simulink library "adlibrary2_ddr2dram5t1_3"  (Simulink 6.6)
libraries: xbsIndex_r4 x5, adlibrary2_ddr2dram5t1_1 x2

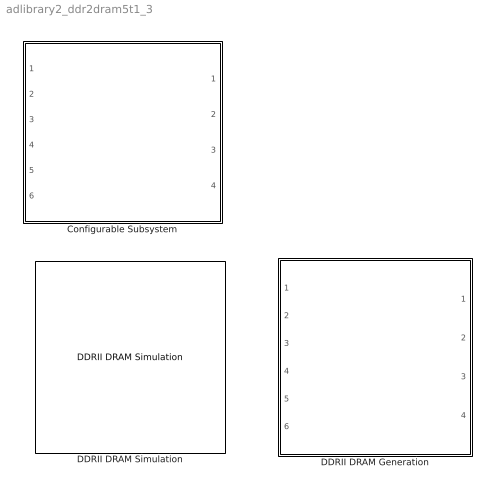
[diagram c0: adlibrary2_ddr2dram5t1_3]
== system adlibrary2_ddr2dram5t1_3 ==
  Configurable Subsystem : Subsystem  BlockChoice=DDRII DRAM Simulation
  DDRII DRAM Generation : Subsystem
  DDRII DRAM Simulation : adlibrary2_ddr2dram5t1_1/DDRII DRAM Simulation  SystemSampleTime=-1

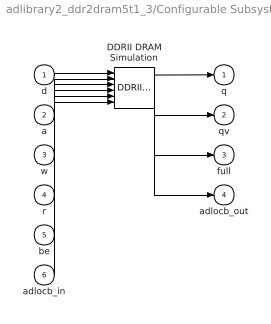
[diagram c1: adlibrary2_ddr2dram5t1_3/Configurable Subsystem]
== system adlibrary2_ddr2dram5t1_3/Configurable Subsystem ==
  d : Inport
  a : Inport  Port=2
  w : Inport  Port=3
  r : Inport  Port=4
  be : Inport  Port=5
  adlocb_in : Inport  Port=6
  DDRII DRAM Simulation : adlibrary2_ddr2dram5t1_1/DDRII DRAM Simulation  SystemSampleTime=-1
  q : Outport
  qv : Outport  Port=2
  full : Outport  Port=3
  adlocb_out : Outport  Port=4
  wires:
  d/1 -> DDRII DRAM Simulation/1
  a/1 -> DDRII DRAM Simulation/2
  w/1 -> DDRII DRAM Simulation/3
  r/1 -> DDRII DRAM Simulation/4
  be/1 -> DDRII DRAM Simulation/5
  adlocb_in/1 -> DDRII DRAM Simulation/6
  DDRII DRAM Simulation/1 -> q/1
  DDRII DRAM Simulation/2 -> qv/1
  DDRII DRAM Simulation/3 -> full/1
  DDRII DRAM Simulation/4 -> adlocb_out/1

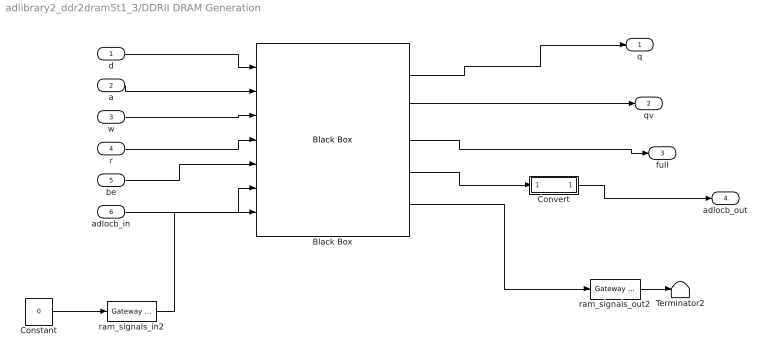
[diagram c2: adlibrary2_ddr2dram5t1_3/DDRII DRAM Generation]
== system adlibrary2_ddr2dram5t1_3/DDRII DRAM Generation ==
  d : Inport
  a : Inport  Port=2
  w : Inport  Port=3
  r : Inport  Port=4
  be : Inport  Port=5
  adlocb_in : Inport  Port=6
  Black Box : xbsIndex_r4/Black Box  init_code=ddr2sdram_v5_config2  sim_method=Inactive  block_type=blackbox2
  Constant : Constant  Value=0
  Convert : Subsystem
  Terminator2 : Terminator
  ram_signals_in2 : xbsIndex_r4/Gateway In  arith_type=Unsigned  n_bits=133  bin_pt=0  quantization="Round  (unbiased: +/- Inf)"  overflow=Saturate  period=ad_get_simulink_period  dbl_ovrd=off  timing_constraint=None  locs_specified=off  LOCs={}  block_type=gatewayin
  ram_signals_out2 : xbsIndex_r4/Gateway Out  hdl_port=on  timing_constraint=None  locs_specified=off  LOCs={}  block_type=gatewayout
  q : Outport
  qv : Outport  Port=2
  full : Outport  Port=3
  adlocb_out : Outport  Port=4
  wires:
  ram_signals_out2/1 -> Terminator2/1
  Constant/1 -> ram_signals_in2/1
  d/1 -> Black Box/1
  a/1 -> Black Box/2
  w/1 -> Black Box/3
  r/1 -> Black Box/4
  be/1 -> Black Box/5
  adlocb_in/1 -> Black Box/6
  Black Box/1 -> q/1
  Black Box/2 -> qv/1
  Black Box/3 -> full/1
  Black Box/4 -> Convert/1(in0)
  Convert/1(out0) -> adlocb_out/1
  ram_signals_in2/1 -> Black Box/7
  Black Box/5 -> ram_signals_out2/1

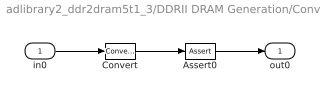
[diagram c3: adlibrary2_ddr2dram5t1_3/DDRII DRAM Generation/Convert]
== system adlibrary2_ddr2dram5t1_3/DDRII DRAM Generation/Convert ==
  in0 : Inport
  Assert0 : xbsIndex_r4/Assert  assert_type=off  type_source=Explicitly  arith_type="Signed  (2's comp)"  n_bits=16  bin_pt=14  assert_rate=on  rate_source=Explicitly  period=ad_get_simulink_period  output_port=on  block_type=assert
  Convert : xbsIndex_r4/Convert  arith_type=Unsigned  n_bits=66  bin_pt=0  quantization=Truncate  overflow=Wrap  latency=0  dbl_ovrd=off  pipeline=off  block_type=convert
  out0 : Outport
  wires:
  in0/1 -> Convert/1
  Convert/1 -> Assert0/1
  Assert0/1 -> out0/1
